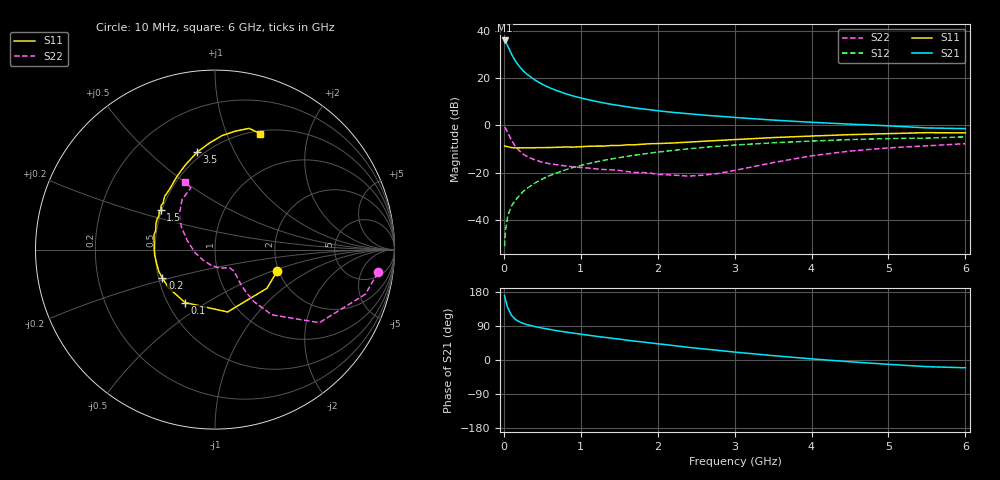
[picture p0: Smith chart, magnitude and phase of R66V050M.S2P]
! SIEMENS Small Signal Semiconductors
! BFR193
! Si NPN RF Bipolar Junction Transistor in SOT23
! VCE = 6 V  IC = 50 mA
! Common Emitter S-Parameters:  May  1996
# GHz  S  MA  R  50
!  f  S11  S21  S12  S22
! GHz  MAG  ANG  MAG  ANG  MAG  ANG  MAG  ANG
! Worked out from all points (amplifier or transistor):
!   36 points, 10 MHz to 6 GHz, reference 50 ohm
!   highest |S21| = 35.9 dB at 10 MHz (marker M1)
!   |S21| within 3 dB of that: start of sweep to 60.54 MHz
!   unconditionally stable (mu >= 1): 420.3 MHz to 1.868 GHz; 1.969 GHz to 2.032 GHz
!   at 250 MHz: K = 0.94, MSG = 25.6 dB, |S12| = -28.0 dB
!   at 1.4 GHz: K = 1.02, MAG = 10.7 dB, |S12| = -14.2 dB
!   at 6 GHz: K = 0.95, MSG = 1.7 dB, |S12| = -4.9 dB
!   S11 on the Smith chart (normalised r, x): 10 MHz: 1.97, -0.54; 100 MHz: 0.61, -0.41; 200 MHz: 0.52, -0.19; 1.5 GHz: 0.49, +0.26; 3.5 GHz: 0.46, +0.72; 6 GHz: 0.53, +1.32
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0.01  0.3671 -18.9  62.29 169.5  0.0028 84.0  0.9162 -8.0
0.02  0.3608 -36.7  59.68 159.9  0.0056 78.0  0.874 -16.5
0.05  0.3545 -78.6  48.11 137.9  0.0121 71.0  0.7099 -35.0
0.1  0.3389 -119.5  31.83 117.7  0.0199 68.5  0.4812 -49.0
0.15  0.3351 -140.5  22.9 107.1  0.0262 68.9  0.3592 -53.3
0.2  0.3333 -151.7  17.75 100.9  0.0327 70.9  0.291 -53.9
0.25  0.3361 -159.0  14.36 96.5  0.0398 72.1  0.247 -53.5
0.3  0.3342 -165.1  12.07 93.4  0.0464 73.8  0.2208 -52.5
0.4  0.337 -174.1  9.191 88.5  0.0599 73.8  0.1872 -50.6
0.5  0.3388 -179.6  7.375 84.2  0.0734 73.5  0.1659 -49.3
0.6  0.3398 175.0  6.186 80.5  0.0873 73.0  0.1542 -49.0
0.7  0.345 170.2  5.344 77.0  0.1008 72.5  0.1464 -49.6
0.8  0.3494 166.3  4.688 73.9  0.1147 71.3  0.1389 -50.2
0.9  0.3469 162.4  4.184 71.0  0.1286 70.1  0.1326 -50.8
1.1  0.3612 155.3  3.482 65.4  0.1556 67.7  0.1252 -55.7
1.5  0.3751 143.6  2.631 55.1  0.2079 62.1  0.1115 -67.4
1.7  0.3887 137.8  2.338 49.8  0.2337 59.3  0.1012 -75.4
2.2  0.4243 125.9  1.881 38.3  0.2956 51.7  0.0891 -105.3
3.5  0.5523 100.4  1.294 11.5  0.4284 31.5  0.1633 161.7
4.5  0.637 86.4  1.062 -4.7  0.5006 17.5  0.2862 133.4
5.5  0.7016 74.3  0.883 -17.6  0.5381 3.9  0.3691 111.4
6  0.6933 68.7  0.854 -20.5  0.572 0.0  0.4109 113.7
